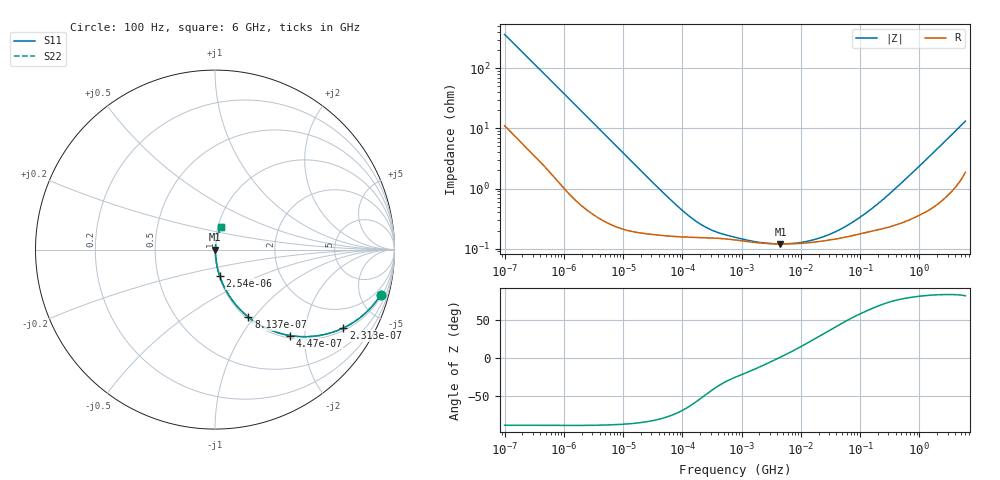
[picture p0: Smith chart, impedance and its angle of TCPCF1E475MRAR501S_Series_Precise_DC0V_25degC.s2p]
! TCPCF1E475MRAR501S Polymer Tantalum Capacitor Sparameter Model
! Model Generated by Samsung Electro-Mechanics
! Samsung Sparameter Version 5.0
! Date : Oct-21-2025
! Products : Polymer Tantalum Capacitor
! Characteristics :
!  Nominal Capacitance = 4.7uF
!  Capacitance Tolerance = +/-20%
!  ESR = 500 mohm max at 100kHz
!  Rated Voltage = 25Vdc
!  Size = 0805(unit:inch), 2012(unit:mm)
!  Length = 2.00+/-0.20mm
!  Width = 1.25+/-0.20mm
!  Thickness = 0.90+/-0.10mm
!  Lineup = Conductive Polymer Type
!  Feature = PCF
!  Measurement Temperature : 25degC.
!  DC bias Value = 0V
!  Frequency : 100Hz ~ 6GHz
! External Node Assignments :
!  1  o---||---o  2
# MHz S RI R 50.0
! Freq.  Real(S11)  Im(S11)  Real(S12)  Im(S12)  Real(S21)  Im(S21)  Real(S22)  Im(S22)
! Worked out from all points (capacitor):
!   300 points, 100 Hz to 6 GHz, reference 50 ohm
!   read as one part in series: C = 4.34 uF near 106.2 Hz
!   lowest |Z| = 120 mohm at 4.534 MHz (marker M1)
!   series resonance near 4.205 MHz, so ESL is about 330 pH
!   S11 on the Smith chart (normalised r, x): 100 Hz: 1.22, -7.29; 231.3 Hz: 1.10, -3.21; 447 Hz: 1.05, -1.68; 813.7 Hz: 1.03, -0.93; 2.54 kHz: 1.01, -0.30; 6 GHz: 1.04, +0.26
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0.0001  0.9236 -0.2509  0.0764 0.2509  0.0764 0.2509  0.9236 -0.2509
0.0001520888  0.8469 -0.3454  0.1531 0.3454  0.1531 0.3454  0.8469 -0.3454
0.00023131  0.7146 -0.437  0.2854 0.437  0.2854 0.437  0.7146 -0.437
0.0004470407  0.4169 -0.4786  0.5831 0.4786  0.5831 0.4786  0.4169 -0.4786
0.0008137405  0.1858 -0.3756  0.8142 0.3756  0.8142 0.3756  0.1858 -0.3756
0.001998454  0.0403 -0.1837  0.9597 0.1837  0.9597 0.1837  0.0403 -0.1837
0.002539509  0.0265 -0.1471  0.9735 0.1471  0.9735 0.1471  0.0265 -0.1471
0.007464481  0.00501 -0.0518  0.995 0.0518  0.995 0.0518  0.00501 -0.0518
0.03993819  0.00177 -0.00989  0.9982 0.00989  0.9982 0.00989  0.00177 -0.00989
0.1041383  0.00157 -0.00386  0.9984 0.00386  0.9984 0.00386  0.00157 -0.00386
0.2012627  0.00153 -0.00204  0.9985 0.00204  0.9985 0.00204  0.00153 -0.00204
0.366355  0.00149 -0.00119  0.9985 0.00119  0.9985 0.00119  0.00149 -0.00119
0.7981464  0.00139 -0.000642  0.9986 0.000642  0.9986 0.000642  0.00139 -0.000642
2.081156  0.00124 -0.000245  0.9988 0.000245  0.9988 0.000245  0.00124 -0.000245
4.534038  0.0012 2.58e-05  0.9988 -2.58e-05  0.9988 -2.58e-05  0.0012 2.58e-05
15.95059  0.00127 0.000561  0.9987 -0.000561  0.9987 -0.000561  0.00127 0.000561
32.7298  0.00141 0.00108  0.9986 -0.00108  0.9986 -0.00108  0.00141 0.00108
63.25518  0.00159 0.00191  0.9984 -0.00191  0.9984 -0.00191  0.00159 0.00191
137.8087  0.0019 0.00371  0.9981 -0.00371  0.9981 -0.00371  0.0019 0.00371
318.7652  0.00236 0.0079  0.9976 -0.0079  0.9976 -0.0079  0.00236 0.0079
1810.813  0.00666 0.0405  0.9933 -0.0405  0.9933 -0.0405  0.00666 0.0405
6000  0.0342 0.1238  0.9658 -0.1238  0.9658 -0.1238  0.0342 0.1238
